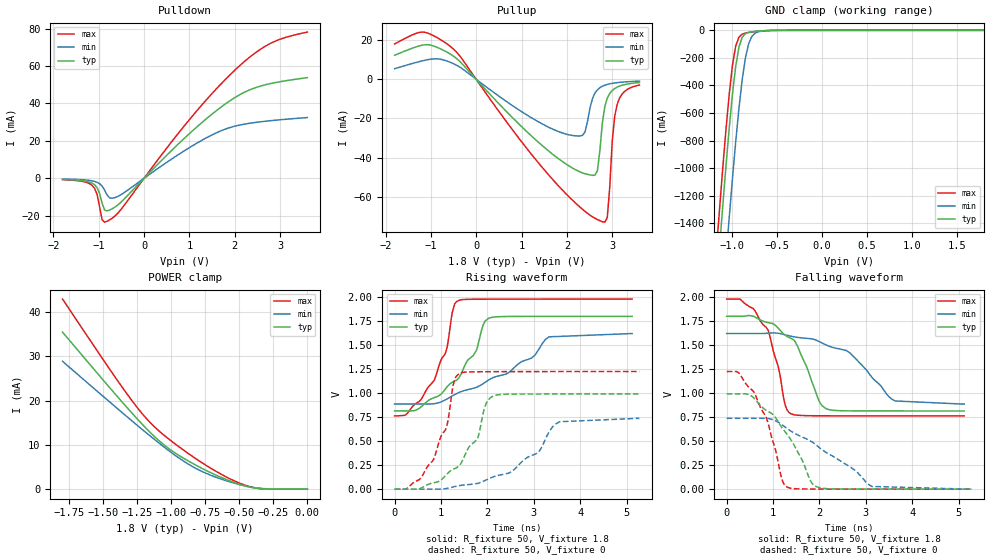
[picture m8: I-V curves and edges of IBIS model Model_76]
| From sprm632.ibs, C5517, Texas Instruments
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| Model based on original model for BC3340CTSCHYPD
|   Sub model SR0_VDD_SR1_VDD_PD_OFF_COM_1P8
[model]   Model_76
|[Description]  [1.8V-I/O-PD_OFF-X, COM]
|   PD_OFF,COM,
|[Input Load]   PD_OFF
|[Output Drive]
|Voltage   1.8V
|Mode   I/O
Model_type   I/O
Polarity   Non-Inverting
Enable   Active-Low
Vinl =  0.63
Vinh =  1.17
Cref =  15.0000pF
Rref =  100.0000M
Vref =  0V
Vmeas =  0.9
C_comp   2.213767p   2.135548p   2.3400939p
[Model Spec]
Vinl   0.63   0.567   0.693
Vinh   1.17   1.053   1.287
[Temperature Range]   25   105   -10
[Voltage Range]   1.8   1.62   1.98
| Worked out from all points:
|   slope of the pulldown table from 0 to 0.27 V, typ, clamps not added: 40.2 ohm
|   slope of the pullup table from 0 to 0.27 V, typ, clamps not added: 39.6 ohm
|   GND clamp passes 1 mA (typ) near -0.58 V on its own axis
|   POWER clamp passes 1 mA (typ) near -0.49 V on its own axis
|   rising waveform, R_fixture 50, V_fixture 1.8: 20-80 % time 803ps typ, 1.58ns min, 555ps max; typ from 0.815 V to 1.8 V
|   rising waveform, R_fixture 50, V_fixture 0: 20-80 % time 680ps typ, 1.05ns min, 504ps max; typ from 0 V to 0.992 V
|   falling waveform, R_fixture 50, V_fixture 1.8: 20-80 % time 659ps typ, 1.08ns min, 460ps max; typ from 1.8 V to 0.814 V
|   falling waveform, R_fixture 50, V_fixture 0: 20-80 % time 766ps typ, 1.44ns min, 505ps max; typ from 0.993 V to 0 V
[POWER_clamp]
-1.8V     35.46mA    28.87mA    42.93mA
-1.455V   22.97mA    19.72mA    27.15mA
-1.273V   16.61mA    14.99mA    19.31mA
-1.145V   12.51mA    11.76mA    14.72mA
-1V       8.751mA    8.276mA    10.88mA
-872.7mV  6.33mA     5.617mA    8.002mA
-763.6mV  4.531mA    3.848mA    5.75mA
-600mV    2.225mA    1.937mA    2.823mA
-472.7mV  845uA      849.5uA    1.055mA
-400mV    327.9uA    407.8uA    392.6uA
-327.3mV  77.63uA    141.5uA    81.87uA
0V        360.5pA    3.06nA     350.8pA
[Pulldown]
-1.8V     -609.1uA   -416.1uA   -761.1uA
-1.364V   -1.277mA   -795.9uA   -1.673mA
-1.145V   -2.657mA   -1.407mA   -3.852mA
-1.036V   -5.115mA   -2.184mA   -8.73mA
-927.3mV  -13.32mA   -4.178mA   -22.18mA
-872.7mV  -16.96mA   -6.282mA   -23.48mA
-763.6mV  -17.01mA   -10.42mA   -22.27mA
-490.9mV  -12.33mA   -8.513mA   -16.08mA
1.036V    24.65mA    16.9mA     32.41mA
1.964V    42.51mA    27.58mA    56.87mA
2.727V    50.26mA    30.59mA    71.28mA
3.6V      53.74mA    32.42mA    78.09mA
[Pullup]
-1.8V     12.32mA    5.441mA    18.09mA
-1.145V   17.63mA    9.682mA    24.11mA
-545.5mV  12.54mA    8.453mA    16.36mA
1.745V    -39.39mA   -26.07mA   -52.75mA
2.345V    -47.87mA   -28.67mA   -66.51mA
2.455V    -48.61mA   -21.59mA   -68.56mA
2.673V    -46.79mA   -5.376mA   -71.69mA
2.836V    -13.94mA   -3.011mA   -73.08mA
2.891V    -9.612mA   -2.61mA    -70.75mA
3V        -5.696mA   -2.054mA   -31.66mA
3.109V    -3.979mA   -1.688mA   -12.82mA
3.6V      -1.642mA   -928.2uA   -2.933mA
[GND_clamp]
-1.8V     -7.733A    -8.408A    -7.463A
-1.182V   -1.913A    -2.609A    -1.63A
-1.145V   -1.597A    -2.289A    -1.316A
-1.109V   -1.289A    -1.974A    -1.014A
-1.036V   -716.9mA   -1.367A    -470.3mA
-1V       -467.4mA   -1.081A    -256.8mA
-963.6mV  -262.8mA   -812.5mA   -115.2mA
-927.3mV  -122.1mA   -568.2mA   -49.46mA
-890.9mV  -50.82mA   -358.8mA   -27.62mA
-818.2mV  -14.85mA   -95.24mA   -15.42mA
-709.1mV  -5.572mA   -10.04mA   -6.496mA
1.8V      360.5pA    6.236uA    -444pA
[Ramp]
dV/dt_f 0.59674854/0.67590621n 0.44445851/1.1170891n 0.73646412/0.47078254n
dV/dt_r 0.59667613/0.68603334n  0.4436906/1.0704964n 0.73629708/0.50662086n
R_load = 50
[Rising Waveform]
R_fixture = 50
V_fixture = 1.8
V_fixture_min = 1.62
V_fixture_max = 1.98
0s        814.9mV    886.9mV    763.6mV
268.6ps   815.3mV    886.9mV    787mV
853.7ps   953.9mV    890.5mV    1.134V
1.095ns   1.044V     930mV      1.416V
1.24ns    1.114V     970.1mV    1.835V
1.356ns   1.145V     999.4mV    1.96V
2.022ns   1.779V     1.135V     1.979V
2.956ns   1.799V     1.366V     1.98V
3.328ns   1.8V       1.587V     1.98V
5.12ns    1.8V       1.62V      1.98V
[Rising Waveform]
R_fixture = 50
V_fixture = 0
V_fixture_min = 0
V_fixture_max = 0
0s        0V         0V         144uV
530.9ps   3.428mV    0V         99.1mV
844.1ps   66.81mV    0V         314.2mV
1.114ns   149.7mV    6.73mV     639.9mV
1.275ns   209.6mV    24.55mV    1.109V
1.394ns   245mV      36.53mV    1.204V
2.144ns   973.1mV    131.5mV    1.224V
3.056ns   991.2mV    370.2mV    1.225V
3.559ns   991.6mV    702.6mV    1.225V
5.277ns   991.9mV    737.1mV    1.225V
[Falling Waveform]
R_fixture = 50
V_fixture = 1.8
V_fixture_min = 1.62
V_fixture_max = 1.98
0s        1.801V     1.621V     1.98V
577.3ps   1.8V       1.621V     1.88V
894.7ps   1.734V     1.625V     1.653V
1.112ns   1.676V     1.623V     1.273V
1.245ns   1.609V     1.609V     906.9mV
1.383ns   1.572V     1.593V     785.8mV
2.143ns   837.7mV    1.502V     763.8mV
2.651ns   815.7mV    1.421V     763.3mV
3.634ns   814.6mV    918.4mV    762.9mV
5.12ns    814.3mV    886.5mV    762.9mV
[Falling Waveform]
R_fixture = 50
V_fixture = 0
V_fixture_min = 0
V_fixture_max = 0
0s        992.6mV    737.8mV    1.225V
264.8ps   992.6mV    737.8mV    1.209V
609.2ps   936.4mV    737.8mV    991.5mV
891ps     809.6mV    735.4mV    692.1mV
1.182ns   646.9mV    674mV      118.8mV
1.297ns   573.8mV    633.5mV    22.95mV
1.801ns   91.81mV    503.2mV    1.548mV
1.989ns   17.38mV    435.6mV    1.139mV
3.133ns   505.3uV    28.16mV    170.9uV
5.277ns   11.04uV    190.8uV    0V
